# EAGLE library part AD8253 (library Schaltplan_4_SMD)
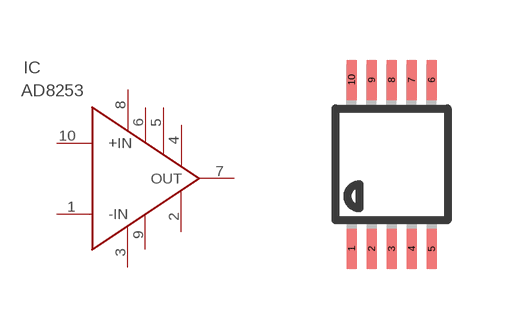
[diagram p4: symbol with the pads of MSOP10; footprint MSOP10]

Designator prefix IC

## AD8253  [MSOP10]
1  -IN  in
2  DGND  pwr
3  -V  pwr
4  A0  in
5  A1  in
6  WR  in
7  OUT  out
8  +V  pwr
9  REF  in
10  +IN  in

## Footprint MSOP10 (pad centres in mm)
10-Lead Mini Small Outline Package [MSOP] (RM-10) Source: http://www.analog.com/UploadedFiles/Data_Sheets/35641221898805SSM2167_b.pdf COMPLIANT TO JEDEC STANDARDS MO-187BA
smd 0.25 x 1: 1 -1,-2.113; 2 -0.5,-2.113; 3 0,-2.113; 4 0.5,-2.113; 5 1,-2.113; 6 1,2.113; 7 0.5,2.113; 8 0,2.113; 9 -0.5,2.113; 10 -1,2.113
